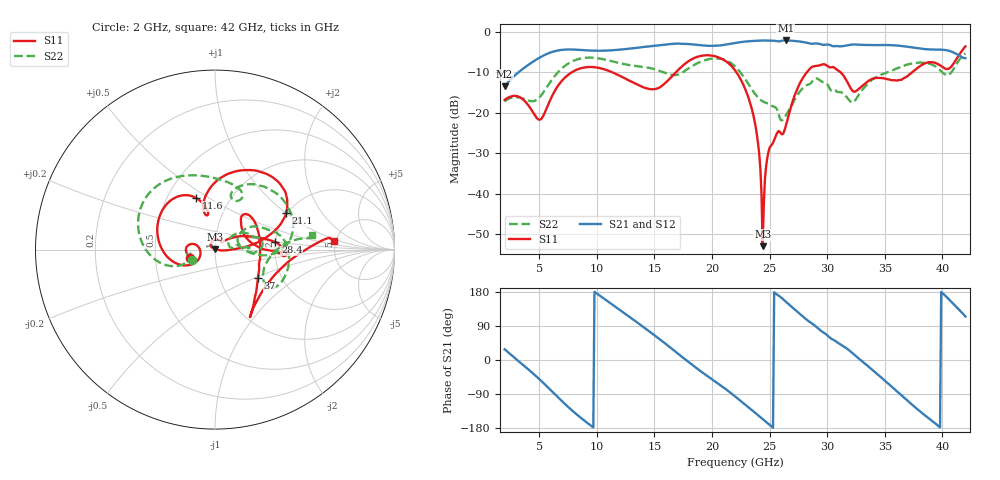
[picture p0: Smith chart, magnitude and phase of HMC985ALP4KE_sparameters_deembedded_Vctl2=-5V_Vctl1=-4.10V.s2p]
!s2p File: Measurements: S11, S21, S12, S22
# GHz S dB R 50.0
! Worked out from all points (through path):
!   401 points, 2 GHz to 42 GHz, reference 50 ohm
!   highest |S21| = -2.08 dB at 26.4 GHz (marker M1); lowest = -13.5 dB at 2 GHz (marker M2)
!   lowest |S11| = -53.0 dB at 24.4 GHz (marker M3), VSWR 1.00, Z = 50.2 + j0.146 ohm
!   |S11| at or under -10 dB: start of sweep to 7.811 GHz; 22.13 GHz to 28.23 GHz (6.097 GHz wide, 24.2 % of centre); 31.17 GHz to 37.36 GHz (6.189 GHz wide, 18.1 % of centre)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
!   |S22| runs from -21.9 to -5.3 dB; largest |S21 - S12| = 0.00082
!   S11 on the Smith chart (normalised r, x): 2 GHz: 0.76, -0.07; 11.6 GHz: 0.69, +0.44; 21.1 GHz: 1.97, +1.00; 28.4 GHz: 2.00, +0.19; 37 GHz: 1.52, -0.53; 42 GHz: 4.82, +0.79
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2  -16.81 -162.0  -13.46 28.3  -13.46 28.3  -17.16 -156.1
5  -21.70 -173.4  -6.39 -50.1  -6.39 -50.1  -16.23 -160.1
6.3  -14.86 -150.9  -4.77 -88.4  -4.77 -88.4  -11.07 -161.6
8.7  -8.91 150.1  -4.45 -154.6  -4.45 -154.6  -6.49 151.3
11.6  -10.28 110.1  -4.46 140.9  -4.46 140.9  -7.42 103.6
13.6  -13.11 100.9  -3.86 97.0  -3.86 97.0  -8.47 76.0
15.4  -13.80 105.6  -3.26 56.2  -3.26 56.2  -9.54 62.6
17.9  -7.33 79.9  -2.96 -3.8  -2.96 -3.8  -9.12 72.2
21.1  -7.02 27.2  -3.15 -74.6  -3.15 -74.6  -6.89 16.0
22  -9.46 16.6  -2.71 -95.9  -2.71 -95.9  -8.51 0.6
23.6  -20.68 -0.1  -2.19 -135.7  -2.19 -135.6  -14.76 -3.6
24  -27.55 -6.7  -2.12 -145.7  -2.12 -145.7  -16.22 2.0
24.4  -53.01 40.7  -2.10 -155.8  -2.10 -155.8  -17.16 7.7
25  -28.70 132.8  -2.13 -171.1  -2.13 -171.1  -17.83 11.1
26.4  -23.36 43.5  -2.08 154.2  -2.08 154.2  -20.69 32.9
28.4  -9.40 7.1  -2.76 102.2  -2.76 102.2  -12.96 18.2
28.7  -8.59 1.9  -2.89 96.1  -2.89 96.1  -12.23 16.5
32.5  -14.62 34.0  -3.10 10.2  -3.10 10.2  -16.63 29.3
35.4  -11.76 18.6  -3.23 -65.2  -3.22 -65.2  -9.78 19.3
37  -10.83 -33.8  -3.65 -108.3  -3.65 -108.2  -8.03 4.9
39.8  -8.23 -56.5  -4.35 -177.8  -4.35 -177.8  -9.42 -34.6
42  -3.55 3.9  -6.44 114.7  -6.45 114.7  -5.28 8.7
